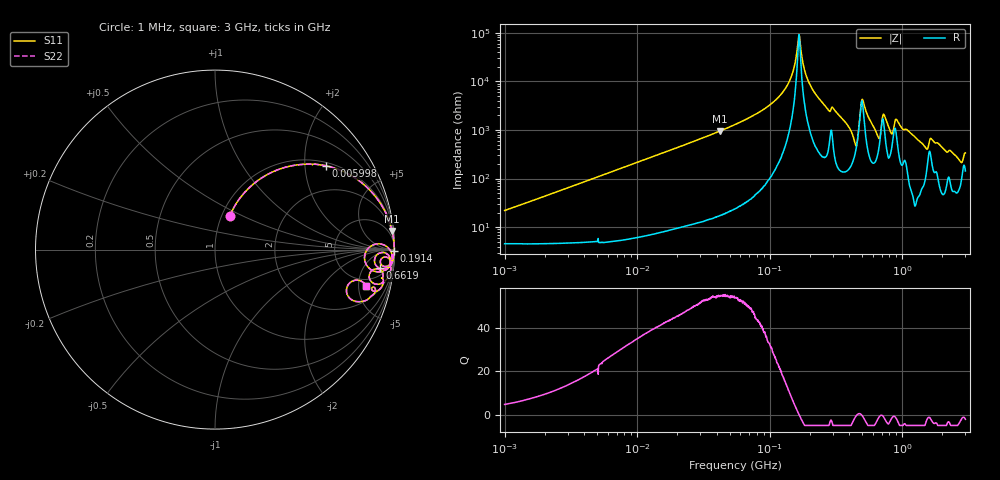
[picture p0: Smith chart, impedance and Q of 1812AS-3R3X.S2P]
!s-Parameter Generated by FASTRON Sdn. Bhd.
!FASTRON P/N : 1812AS-3R3X
!Keysight Technologies,E4991B,MY54100416,A.01.15
!Date created: Fri Oct 13 15:54:47 2023
!Version  : Rev00 Fri Oct 13 15:54:47 2023
!Data & Calibration Information:
!Freq	S11	S21	S12	S22
!PortZ  Port1:50+j0  Port2:50+j0
!When reading, reference impedance value at option line is always used.
! Remarks : This data is being provided solely for informational purposes.
# Hz S dB R 50
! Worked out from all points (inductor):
!   1601 points, 1 MHz to 3 GHz, reference 50 ohm
!   read as one part in series: L = 3.43 uH near 1.041 MHz
!   highest Q = 55.1 at 42.01 MHz (marker M1), where L = 3.58 uH
!   self-resonance near 166.3 MHz
!   S11 on the Smith chart (normalised r, x): 1 MHz: 1.09, +0.43; 5.998 MHz: 1.10, +2.58; 191.4 MHz: open; 661.9 MHz: 8, -12; 3 GHz: 3.87, -6.12
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1000000  -13.71 66.4  -0.57 -11.6  -0.57 -11.6  -13.71 66.4
3804036  -4.21 48.7  -2.47 -37.9  -2.47 -37.9  -4.21 48.7
5997992  -2.21 37.0  -4.41 -50.8  -4.41 -50.8  -2.21 37.0
1.447069e7  -0.49 17.7  -10.34 -70.9  -10.34 -70.9  -0.49 17.7
4.201274e7  -0.06 6.0  -19.59 -82.9  -19.59 -82.9  -0.06 6.0
5.477226e7  -0.04 4.4  -22.26 -84.5  -22.26 -84.5  -0.04 4.4
1.238204e8  -0.01 1.0  -35.13 -85.9  -35.13 -85.9  -0.01 1.0
1.467848e8  -0.01 0.4  -42.44 -82.2  -42.44 -82.2  -0.01 0.4
1.663456e8  -0.01 0.0  -59.30 -5.7  -59.30 -5.7  -0.01 0.0
1.913643e8  -0.01 -0.5  -41.44 81.3  -41.44 81.3  -0.01 -0.5
2.083556e8  -0.01 -0.8  -37.14 83.7  -37.14 83.7  -0.01 -0.8
4.413523e8  -1.03 -7.6  -15.50 44.6  -15.50 44.6  -1.03 -7.6
5.051982e8  -0.16 -0.9  -32.44 41.0  -32.44 41.0  -0.16 -0.9
6.619339e8  -0.70 -6.5  -17.53 51.4  -17.53 51.4  -0.70 -6.5
7.279565e8  -0.26 -2.1  -26.64 49.9  -26.64 49.9  -0.26 -2.1
7.925923e8  -0.21 -4.9  -21.19 71.5  -21.19 71.5  -0.21 -4.9
8.332625e8  -0.55 -5.6  -18.99 54.2  -18.99 54.2  -0.55 -5.6
9.117997e8  -0.23 -3.2  -24.36 63.1  -24.36 63.1  -0.23 -3.2
1.496395e9  -0.63 -12.0  -13.43 65.1  -13.43 65.1  -0.63 -12.0
1.662201e9  -0.54 -7.7  -16.90 61.3  -16.90 61.3  -0.54 -7.7
2.714296e9  -1.48 -20.1  -8.95 54.3  -8.95 54.3  -1.48 -20.1
3e9  -1.27 -13.4  -11.85 51.5  -11.85 51.5  -1.27 -13.4
